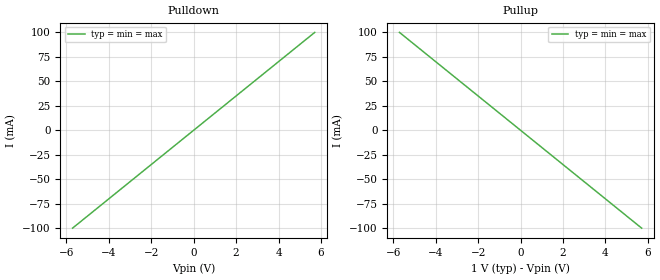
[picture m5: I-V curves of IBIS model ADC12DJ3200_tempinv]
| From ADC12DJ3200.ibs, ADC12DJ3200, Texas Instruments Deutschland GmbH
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[Model] ADC12DJ3200_tempinv
Model_type Output
C_comp   0   0   0
Cref = 0
Vref = 0.5
Rref = 50
Vmeas = 0.5
[Temperature_Range] 25 125 0
[Voltage Range]  1  1  1
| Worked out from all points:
|   slope of the pulldown table from 0 to 0.15 V, typ, clamps not added: 57.1 ohm
|   slope of the pullup table from 0 to 0.15 V, typ, clamps not added: 57.1 ohm
[Pulldown]
-5.706V   -100mA     -100mA     -100mA
0V        0A         0A         0A
5.706V    100mA      100mA      100mA
[Pullup]
-5.706V   100mA      100mA      100mA
0V        0A         0A         0A
5.706V    -100mA     -100mA     -100mA
[Ramp]
dV/dt_r 0.2/1p 0.2/1p 0.2/1p
dV/dt_f 0.2/1p 0.2/1p 0.2/1p
[Algorithmic Model]
Executable Windows_cl19.00.24215.1_64 ADC12DJ3200_x64.dll ADC12DJ3200_tempinv.ami
Executable Linux_gcc4.7.4_64 ADC12DJ3200_x64.so ADC12DJ3200_tempinv.ami
[End Algorithmic Model]
